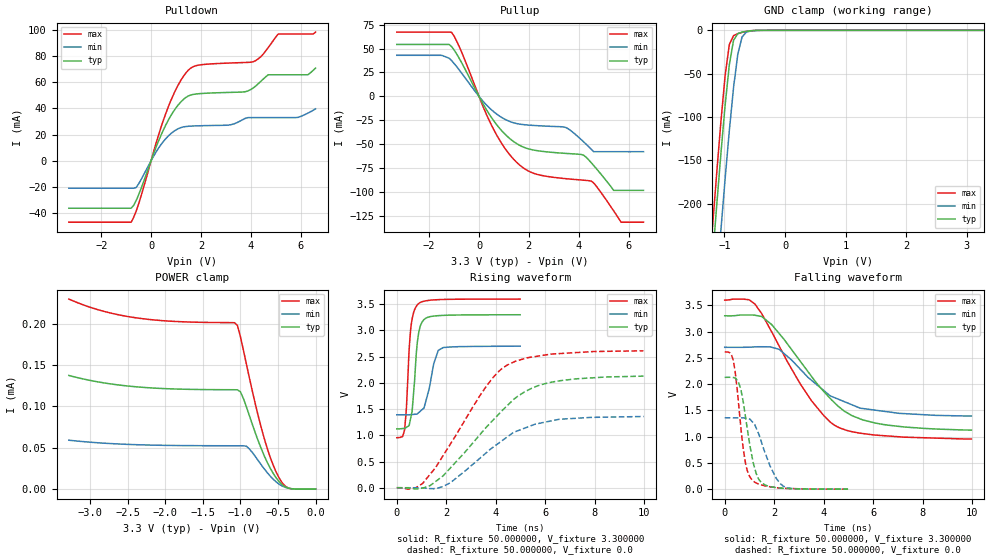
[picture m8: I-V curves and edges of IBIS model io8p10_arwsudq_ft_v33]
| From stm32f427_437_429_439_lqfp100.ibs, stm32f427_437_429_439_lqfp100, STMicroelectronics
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|   Model io8p10_arwsudq_ft_v33
[Model]  io8p10_arwsudq_ft_v33
Model_type I/O
Polarity   Non-Inverting
Enable   Active-Low
Vinl =   0.990000V
Vinh =   2.310000V
Vmeas =  1.650000V
Cref =   40.000000pF
Rref =   100.000000M
Vref =   0.0V
C_comp   2.911600pF   2.823500pF   2.988000pF
[Temperature Range]   25.000000   0.125000k   -40.000000
[Pullup Reference]   3.300000V   2.700000V   3.600000V
[Pulldown Reference]   0.0V   0.0V   0.0V
[POWER Clamp Reference]   3.300000V   2.700000V   3.600000V
[GND Clamp Reference]   0.0V   0.0V   0.0V
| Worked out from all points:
|   slope of the pulldown table from 0 to 0.495 V, typ, clamps not added: 20.9 ohm
|   slope of the pullup table from 0 to 0.495 V, typ, clamps not added: 22.6 ohm
|   GND clamp passes 1 mA (typ) near -0.62 V on its own axis
|   rising waveform, R_fixture 50.000000, V_fixture 3.300000: 20-80 % time 220ps typ, 369ps min, 189ps max; typ from 1.12 V to 3.3 V
|   rising waveform, R_fixture 50.000000, V_fixture 0.0: 20-80 % time 2.51ns typ, 2.26ns min, 2.12ns max; typ from 0 V to 2.13 V
|   falling waveform, R_fixture 50.000000, V_fixture 3.300000: 20-80 % time 2.26ns typ, 2.15ns min, 2.05ns max; typ from 3.3 V to 1.12 V
|   falling waveform, R_fixture 50.000000, V_fixture 0.0: 20-80 % time 465ps typ, 673ps min, 372ps max; typ from 2.13 V to 0 V
[Pulldown]
|Voltage   I(typ)   I(min)   I(max)
-3.3V     -36.38mA   -21.07mA   -47.08mA
-800mV    -36.38mA   -21.07mA   -47.08mA
-600mV    -30.5mA    -20.54mA   -38.69mA
700mV     31.4mA     19.11mA    41.71mA
1.2V      45.15mA    25.37mA    61.75mA
1.6V      50.35mA    26.5mA     71.06mA
3.1V      52.28mA    27.26mA    74.76mA
4.1V      55.71mA    33.02mA    75.8mA
4.7V      65.8mA     33.02mA    86.64mA
5.1V      65.8mA     33.02mA    97.03mA
6.3V      65.87mA    36.5mA     97.03mA
6.6V      70.93mA    39.72mA    98.49mA
[Pullup]
|Voltage   I(typ)   I(min)   I(max)
-3.3V     54.21mA    42.91mA    67.14mA
-1.5V     54.21mA    42.91mA    67.14mA
-1.1V     51.97mA    37.28mA    66.86mA
500mV     -22.07mA   -14mA      -30.03mA
1.5V      -49.1mA    -28.3mA    -68.56mA
2.2V      -56.05mA   -30.32mA   -80.35mA
3.5V      -59.53mA   -32.66mA   -85.92mA
4.2V      -61.45mA   -47.47mA   -87.46mA
4.5V      -69.1mA    -55.02mA   -88.4mA
5.4V      -98.1mA    -57.7mA    -119.3mA
5.7V      -98.1mA    -57.7mA    -131.3mA
6.6V      -98.1mA    -57.7mA    -131.3mA
[GND_clamp]
|Voltage   I(typ)   I(min)   I(max)
-3.3V     -2.32A     -2.397A    -2.297A
-1.2V     -266.4mA   -356.3mA   -229.4mA
-1.13V    -203.6mA   -293.1mA   -166.3mA
-1.06V    -143.2mA   -231.4mA   -106.2mA
-990mV    -86.95mA   -171.8mA   -52.65mA
-920mV    -39.66mA   -115.8mA   -16.36mA
-850mV    -11.49mA   -65.84mA   -6.11mA
-780mV    -3.834mA   -27.59mA   -3.88mA
-710mV    -2.09mA    -7.753mA   -2.381mA
-640mV    -1.147mA   -2.129mA   -1.22mA
-570mV    -523.9uA   -800uA     -476.8uA
3.28V     0A         0A         0A
[POWER_clamp]
|Voltage   I(typ)   I(min)   I(max)
-3.28V    137.3uA    59.14uA    229.6uA
-2.36V    123.4uA    53.65uA    206.6uA
-1.08V    120.1uA    52.41uA    201.1uA
-1.04V    120uA      52.41uA    198uA
-1V       117.7uA    52.4uA     184.5uA
-920mV    99.46uA    51.91uA    151.2uA
-720mV    48.42uA    29.12uA    73.51uA
-600mV    24.82uA    15.47uA    37.72uA
-520mV    13.1uA     8.45uA     19.84uA
-440mV    5.058uA    3.61uA     7.276uA
-360mV    1.193uA    1.129uA    1.311uA
0V        0A         0A         0A
[Ramp]
| variable   typ   min   max
dV/dt_r  1.26942/2.51658n   0.81204/2.26120n   1.56522/2.11977n
dV/dt_f  1.28538/2.25290n   0.77832/2.14974n   1.57597/2.04865n
R_load = 50.000000
[Rising Waveform]
R_fixture= 50.000000
V_fixture= 3.300000
V_fixture_min= 2.700000
V_fixture_max= 3.600000
|time   V(typ)   V(min)   V(max)
0s        1.124V     1.392V     954.2mV
320.3ps   1.132V     1.392V     1.121V
390.4ps   1.153V     1.391V     1.529V
500.5ps   1.187V     1.391V     2.641V
620.6ps   1.464V     1.397V     3.219V
850.9ps   2.844V     1.418V     3.499V
1.101ns   3.208V     1.522V     3.558V
1.491ns   3.274V     2.363V     3.583V
1.682ns   3.282V     2.623V     3.588V
4.985ns   3.3V       2.7V       3.599V
[Rising Waveform]
R_fixture= 50.000000
V_fixture= 0.0
V_fixture_min= 0.0
V_fixture_max= 0.0
|time   V(typ)   V(min)   V(max)
0s        198.3uV    84.7uV     715uV
560.6ps   -10.43mV   -60.29uV   -21.75mV
1.041ns   -5.67mV    -4.936mV   80.86mV
1.361ns   45.48mV    -16.25mV   265mV
2.182ns   385.8mV    100.6mV    844.5mV
3.604ns   1.147V     661.8mV    1.925V
4.444ns   1.557V     962.7mV    2.334V
5.185ns   1.834V     1.14V      2.467V
6.186ns   2.007V     1.27V      2.546V
9.97ns    2.129V     1.359V     2.612V
[Falling Waveform]
R_fixture= 50.000000
V_fixture= 3.300000
V_fixture_min= 2.700000
V_fixture_max= 3.600000
|time   V(typ)   V(min)   V(max)
0s        3.3V       2.7V       3.599V
981ps     3.315V     2.702V     3.605V
1.221ns   3.31V      2.708V     3.523V
1.502ns   3.284V     2.711V     3.336V
2.202ns   2.962V     2.661V     2.723V
3.504ns   2.15V      2.074V     1.685V
4.464ns   1.633V     1.737V     1.21V
5.145ns   1.4V       1.605V     1.093V
6.066ns   1.261V     1.505V     1.03V
9.97ns    1.124V     1.392V     954.2mV
[Falling Waveform]
R_fixture= 50.000000
V_fixture= 0.0
V_fixture_min= 0.0
V_fixture_max= 0.0
|time   V(typ)   V(min)   V(max)
0s        2.129V     1.359V     2.612V
340.3ps   2.125V     1.358V     2.461V
560.6ps   2.032V     1.358V     1.63V
680.7ps   1.834V     1.357V     1.046V
840.8ps   1.376V     1.35V      494mV
1.091ns   651.6mV    1.295V     187.3mV
1.451ns   143mV      944.9mV    85.38mV
1.832ns   50.23mV    442.3mV    45.24mV
2.362ns   17.7mV     60.23mV    16.76mV
4.985ns   198.3uV    84.7uV     715uV
